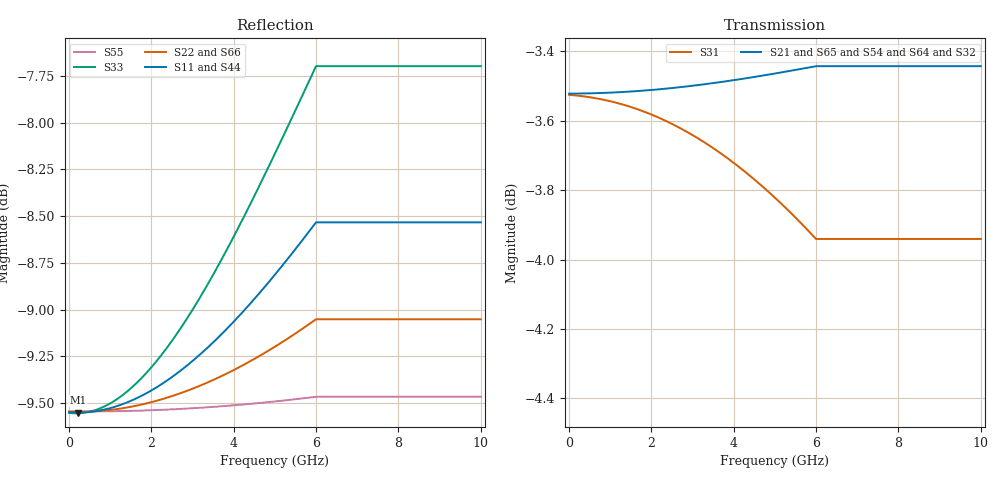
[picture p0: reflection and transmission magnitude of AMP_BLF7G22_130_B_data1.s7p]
! Created Thu Jul 08 13:22:21 2010
# ghz S ma R 50
! 7 Port Network Data from SP1.SP block
! freq  magS11  angS11  magS12  angS12  magS13  angS13  magS14  angS14
!  magS15  angS15  magS16  angS16  magS17  angS17
!  magS21  angS21
!  magS22  angS22  magS23  angS23  magS24  angS24  magS25  angS25
!  magS26  angS26  magS27  angS27
!  magS31  angS31  magS32  angS32
!  magS33  angS33  magS34  angS34  magS35  angS35  magS36  angS36
!  magS37  angS37
!  magS41  angS41  magS42  angS42  magS43  angS43
!  magS44  angS44  magS45  angS45  magS46  angS46  magS47  angS47
!  magS51  angS51  magS52  angS52  magS53  angS53  magS54  angS54
!  magS55  angS55  magS56  angS56  magS57  angS57
!  magS61  angS61
!  magS62  angS62  magS63  angS63  magS64  angS64  magS65  angS65
!  magS66  angS66  magS67  angS67
!  magS71  angS71  magS72  angS72
!  magS73  angS73  magS74  angS74  magS75  angS75  magS76  angS76
!  magS77  angS77
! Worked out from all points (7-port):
!   1000 points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, 10 MHz to 10 GHz, reference 50 ohm
!   strongest paths, dB at 10 MHz, 2.51 GHz, 5.01 GHz, 7.51 GHz, 10 GHz:
!     S21: -3.5, -3.5, -3.5, -3.4, -3.4
!     S65: -3.5, -3.5, -3.5, -3.5, -3.5
!     S54: -3.5, -3.5, -3.6, -3.6, -3.6
!     S64: -3.5, -3.6, -3.6, -3.7, -3.7
!     S32: -3.5, -3.6, -3.7, -3.8, -3.8
!     S31: -3.5, -3.6, -3.8, -3.9, -3.9
!   lowest |S11| = -9.6 dB at 220 MHz (marker M1), VSWR 2.00, Z = 25 + j0.571 ohm
!   |S11| at or under -10 dB: nowhere
